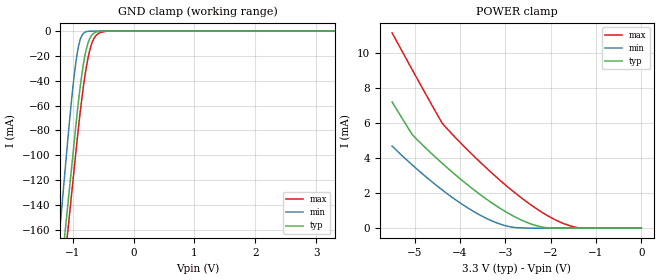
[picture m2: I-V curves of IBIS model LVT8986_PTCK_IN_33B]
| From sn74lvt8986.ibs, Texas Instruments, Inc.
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[Model]   LVT8986_PTCK_IN_33B
Model_type  Input
Vinl=0.8
Vinh=2.0
| variable   typ   min   max
C_comp   3.18pF   2.51pF   4.49pF
[Temperature Range]   40   -40   100
| Ambient temperature   25   -40   85
[Voltage range]   3.3   2.7   3.6
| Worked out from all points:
|   GND clamp passes 1 mA (typ) near -0.62 V on its own axis
|   POWER clamp passes 1 mA (typ) near -3.03 V on its own axis
[GND Clamp]
| LVT8986_PTCK_IN_33B
|   Voltage   I(typ)   I(min)   I(max)
-5.5V     -2.287A    -2.545A    -2.286A
-1.225V   -210.7mA   -168.1mA   -231.2mA
-1.195V   -196.2mA   -151.4mA   -216.8mA
-1.135V   -167.1mA   -118.2mA   -188mA
-1.105V   -152.6mA   -101.6mA   -173.6mA
-1.075V   -138.1mA   -84.99mA   -159.2mA
-975mV    -89.68mA   -35.99mA   -111.2mA
-900mV    -54.92mA   -11.37mA   -75.86mA
-775mV    -14.49mA   -464.5uA   -29.03mA
-700mV    -4.239mA   -23.21uA   -12.06mA
-600mV    -600.8uA   -202.5nA   -2.821mA
3.3V      16.16pA    8.099pA    391.9pA
[POWER Clamp]
| LVT8986_PTCK_IN_33B
|   Voltage   I(typ)   I(min)   I(max)
-5.5V     7.191mA    4.679mA    11.13mA
-5.055V   5.335mA    3.603mA    9.023mA
-4.39V    3.688mA    2.171mA    5.968mA
-3.895V   2.595mA    1.261mA    4.615mA
-3.45V    1.713mA    598.2uA    3.501mA
-3.055V   1.033mA    183.2uA    2.585mA
-2.715V   547.5uA    22.73uA    1.862mA
-2.17V    55.3uA     4.609nA    869.2uA
-1.83V    1.773uA    13.4pA     391.7uA
-1.525V   8.748nA    11.66pA    99.72uA
-1.26V    91.77pA    10.63pA    5.075uA
-95.1fV   16.16pA    5.854pA    469.5pA
